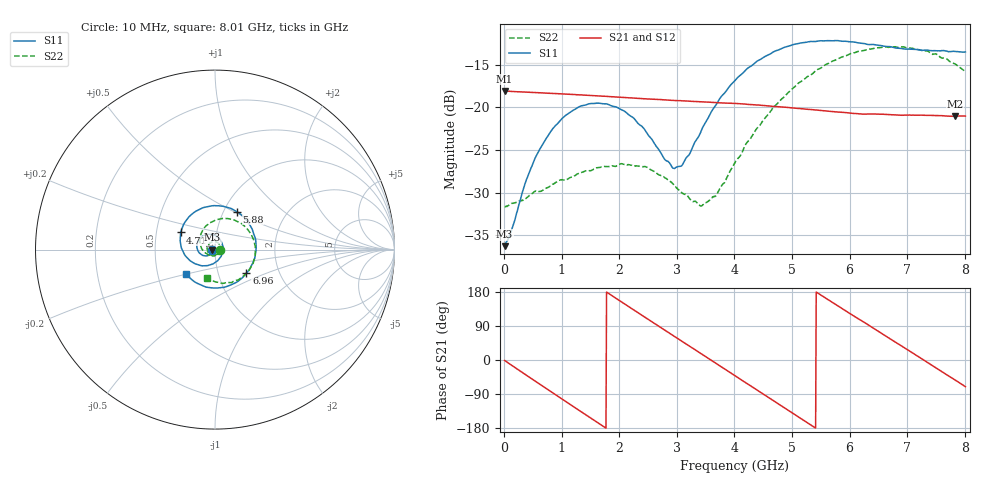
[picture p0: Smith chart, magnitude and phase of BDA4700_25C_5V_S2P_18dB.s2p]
!Agilent Technologies,E5071B,MY42404982,A.09.10
!Date: Mon Oct 20 13:35:19 2025
!Data & Calibration Information:
!Freq	S11:SOLT2(ON)	S21:SOLT2(ON)	S12:SOLT2(ON)	S22:SOLT2(ON)
# Hz S RI R 50
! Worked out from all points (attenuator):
!   801 points, 10 MHz to 8.01 GHz, reference 50 ohm
!   highest |S21| = -18.09 dB at 10 MHz (marker M1); lowest = -21.1 dB at 7.83 GHz (marker M2)
!   lowest |S11| = -36.3 dB at 10 MHz (marker M3), VSWR 1.03, Z = 48.5 - j0.123 ohm
!   |S11| at or under -10 dB: start of sweep to end of sweep
!   |S22| runs from -31.7 to -12.9 dB; largest |S21 - S12| = 0.00089
!   S11 on the Smith chart (normalised r, x): 10 MHz: 0.97, -0.00; 4.71 GHz: 0.67, +0.13; 5.88 GHz: 1.15, +0.52; 6.96 GHz: 1.36, -0.38; 8.01 GHz: 0.70, -0.20
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1e7  -0.0153 -0.00126  0.1246 -0.00274  0.1246 -0.0028  0.0262 -0.000857
1.4e8  -0.0167 -0.00999  0.1195 -0.0314  0.1195 -0.0315  0.0265 -0.0069
3.9e8  -0.0269 -0.0265  0.0934 -0.0793  0.0934 -0.0794  0.0209 -0.0207
6e8  -0.0428 -0.0348  0.0577 -0.107  0.0575 -0.1071  0.0122 -0.0296
1e9  -0.0819 -0.0237  -0.0253 -0.1169  -0.0254 -0.1171  -0.0162 -0.0339
1.35e9  -0.1013 0.0123  -0.0871 -0.0796  -0.0871 -0.0796  -0.0381 -0.0164
2.07e9  -0.0442 0.0848  -0.0991 0.0567  -0.0991 0.0567  -0.0282 0.0367
2.68e9  0.0353 0.0444  0.000513 0.111  0.000498 0.111  0.0179 0.0361
2.93e9  0.0438 0.00386  0.0463 0.0995  0.0463 0.0993  0.0287 0.021
3.06e9  0.041 -0.0187  0.067 0.0862  0.0665 0.0865  0.0304 0.01
3.43e9  -0.00205 -0.0736  0.1036 0.0293  0.1036 0.0293  0.0184 -0.019
3.69e9  -0.0535 -0.0897  0.1048 -0.0181  0.1049 -0.0184  -0.0028 -0.0306
4.01e9  -0.1243 -0.0712  0.0788 -0.0697  0.0788 -0.0696  -0.0376 -0.0284
4.71e9  -0.1912 0.0953  -0.036 -0.0943  -0.0357 -0.0945  -0.085 0.0571
5.35e9  -0.0566 0.236  -0.0962 -0.0104  -0.0962 -0.0106  -0.0131 0.1561
5.88e9  0.121 0.2115  -0.0656 0.0663  -0.0655 0.0662  0.1118 0.1628
6.26e9  0.2083 0.1105  -0.0138 0.0899  -0.013 0.09  0.1911 0.0995
6.68e9  0.2226 -0.0417  0.0478 0.0768  0.048 0.0768  0.2243 -0.0102
6.96e9  0.1749 -0.1323  0.0766 0.047  0.0767 0.0466  0.207 -0.0871
7.38e9  0.0432 -0.2106  0.0884 -0.0144  0.0885 -0.0145  0.1244 -0.1697
7.83e9  -0.115 -0.1786  0.0537 -0.0703  0.0537 -0.0705  0.0005 -0.1793
8.01e9  -0.1624 -0.1344  0.0298 -0.0836  0.03 -0.0836  -0.0419 -0.1557
